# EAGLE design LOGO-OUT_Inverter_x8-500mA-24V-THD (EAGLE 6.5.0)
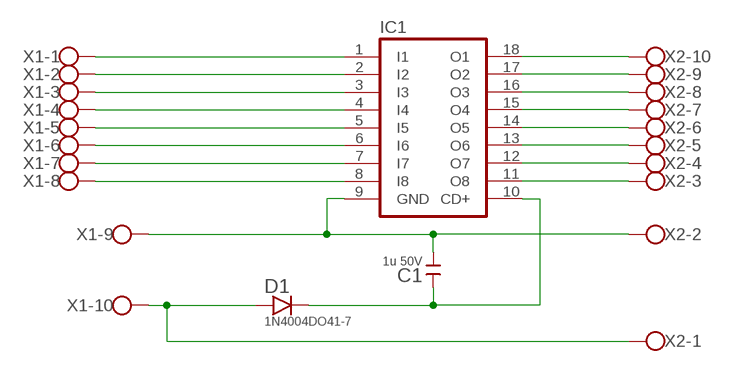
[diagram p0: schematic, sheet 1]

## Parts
C1  1u 50V  C-EU025-024X044  [C025-024X044]
D1  1N4004DO41-7  [DO41-7]
IC1  ULN2803A  [DIL18]
X1  AK500/10  [AK500/10]
X2  AK500/10  [AK500/10]

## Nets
N$1: IC1.1(I1) X1.1
N$2: IC1.2(I2) X1.2
N$3: IC1.3(I3) X1.3
N$4: IC1.4(I4) X1.4
N$5: IC1.5(I5) X1.5
N$6: IC1.6(I6) X1.6
N$7: IC1.7(I7) X1.7
N$8: IC1.8(I8) X1.8
N$9: D1.A X1.10 X2.1
N$10: C1.2 IC1.9(GND) X1.9 X2.2
N$11: IC1.18(O1) X2.10
N$12: IC1.17(O2) X2.9
N$13: IC1.16(O3) X2.8
N$14: IC1.15(O4) X2.7
N$15: IC1.14(O5) X2.6
N$16: IC1.13(O6) X2.5
N$17: IC1.12(O7) X2.4
N$18: IC1.11(O8) X2.3
N$19: C1.1 D1.C IC1.10(CD+)

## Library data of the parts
C1 = rcl:C-EU: CAPACITOR, European symbol
D1 = diode:1N4004: DIODE
IC1 = uln-udn:ULN2803A: DRIVER ARRAY
X1 X2 = con-ptr500:AK500/10: CONNECTOR

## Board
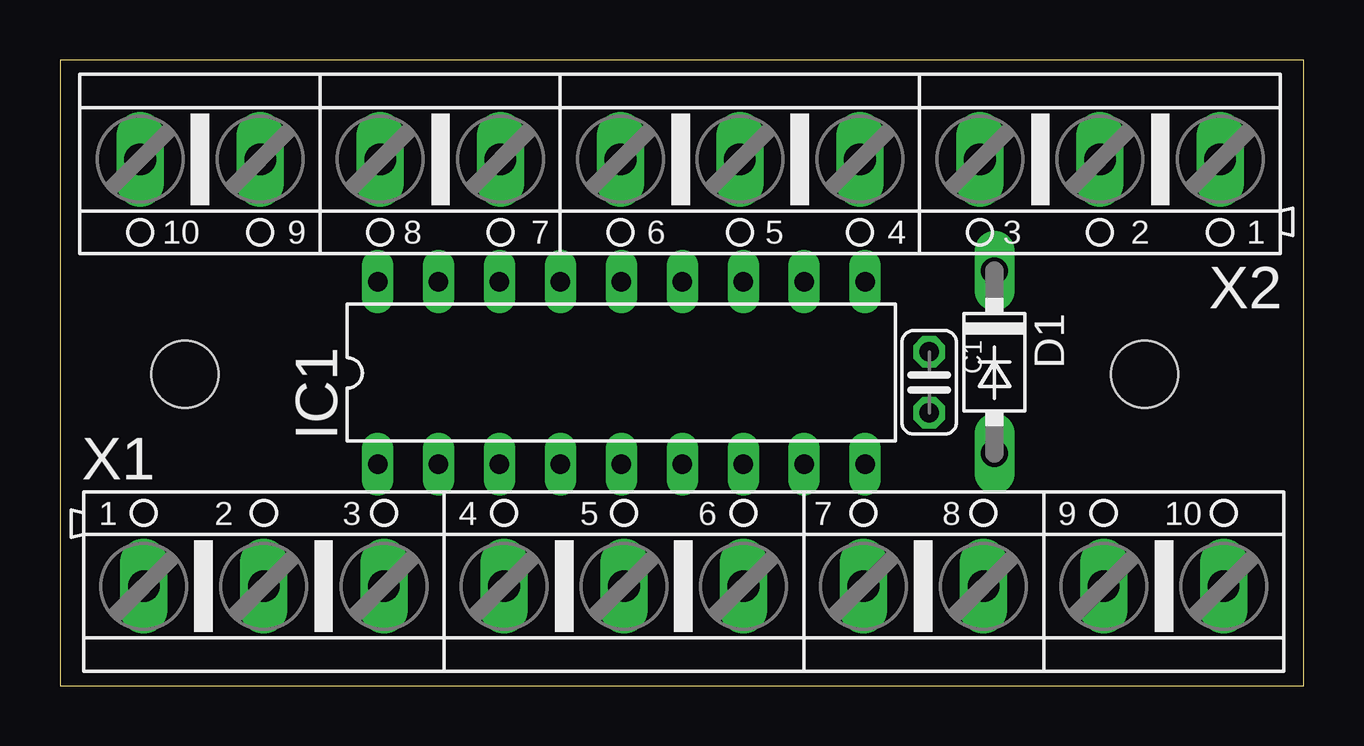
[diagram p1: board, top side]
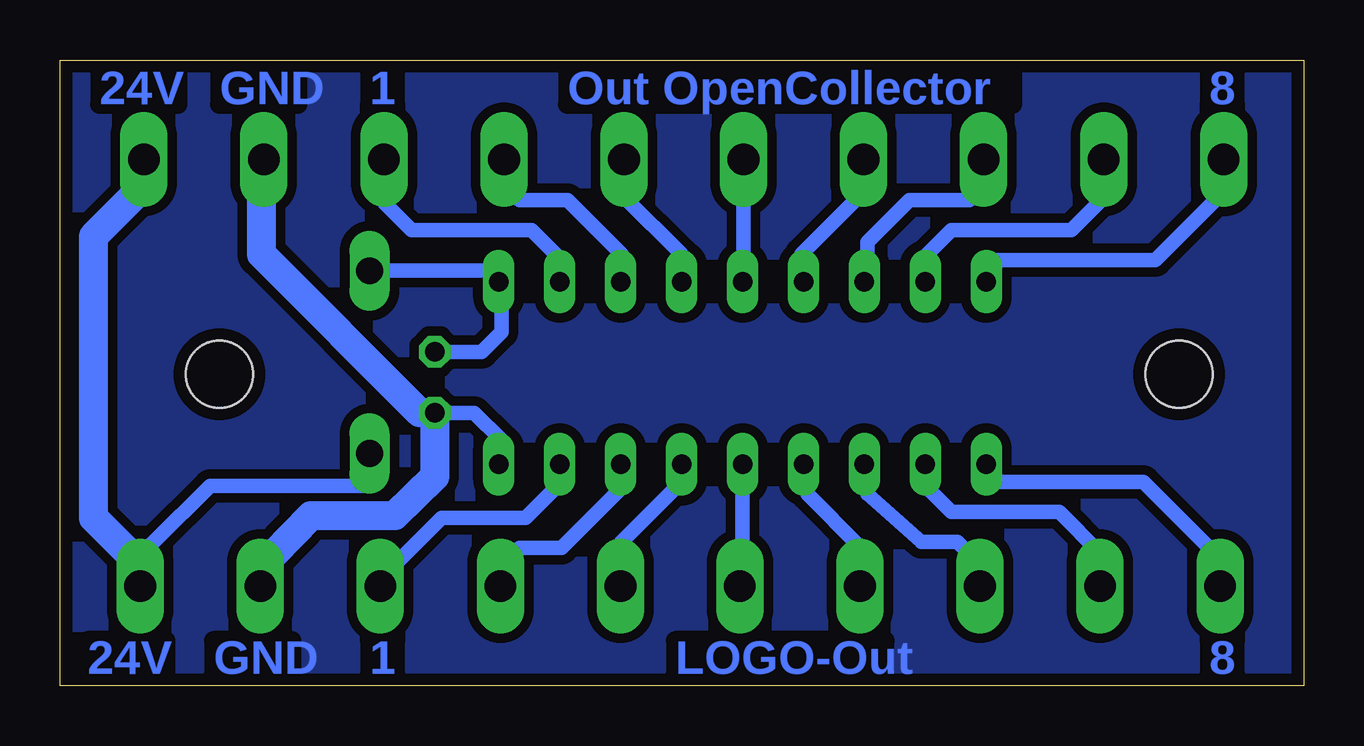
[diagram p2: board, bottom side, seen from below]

Size 51.85 x 26.1 mm. Coordinates in mm from the lower left corner, seen from the top.
Outline: 51.85,0 51.85,26.1 0,26.1 0,0 51.85,0
Copper layers ((1*2)+(15*16)): Top 0.035mm / dielectric 0.7mm / Route2 0.035mm / dielectric 0.15mm / Route15 0.035mm / dielectric 0.7mm / Bottom 0.035mm
Design rules "default *": minimum track width 0.6mm, minimum drill 0.3mm, track to track 0.15mm, track to pad 0.15mm, pad to pad 0.15mm, via to via 0.15mm, smd to smd 2mil, copper to edge 20mil, drill to drill 7mil, minimum pad ring 10mil, minimum via ring 8mil, stop-mask expansion 0.05mm, vias tented up to drill 0.6mm, thermal gap 10mil
Holes 2.8 mm at 5.2,13 45.2,13

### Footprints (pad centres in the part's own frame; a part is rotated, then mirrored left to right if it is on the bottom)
C025-024X044 = drill 0.813 octagon: 1 -1.27,0; 2 1.27,0
DO41-7 = drill 1.118 long: A 3.81,0; C -3.81,0
DIL18 = drill 0.813 long: 1 -10.16,-3.81; 2 -7.62,-3.81; 3 -5.08,-3.81; 4 -2.54,-3.81; 5 0,-3.81; 6 2.54,-3.81; 7 5.08,-3.81; 8 7.62,-3.81; 9 10.16,-3.81; 10 10.16,3.81; 11 7.62,3.81; 12 5.08,3.81; 13 2.54,3.81; 14 0,3.81; 15 -2.54,3.81; 16 -5.08,3.81; 17 -7.62,3.81; 18 -10.16,3.81
AK500/10 = drill 1.321 long: 1 -22.504,0; 2 -17.501,0; 3 -12.497,0; 4 -7.493,0; 5 -2.489,0; 6 2.489,0; 7 7.493,0; 8 12.497,0; 9 17.501,0; 10 22.504,0

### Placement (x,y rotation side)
C1  36.23,12.66 270 top
D1  38.95,13.5 270 top
IC1  23.4,13.05 0 top
X1  26,4.16 0 top
X2  25.85,21.96 180 top

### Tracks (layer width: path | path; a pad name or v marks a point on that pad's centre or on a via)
N$1
  Bottom 0.6: X1.1 3.5,5.3 6.7,8.5 13.25,8.5 IC1.1
N$2
  Bottom 0.6: X1.2 8.5,5.55 10.2,7.25 14.7,7.25 15.7,8.25 15.7,9.16 IC1.2
N$3
  Bottom 0.6: X1.3 13.5,5.05 14.45,6 15.95,6 18.2,8 18.2,9.12 IC1.3
N$4
  Bottom 0.6: X1.4 18.51,5.81 20.7,8 20.7,9.08 IC1.4
N$5
  Bottom 0.6: IC1.5 23.4,4.27 X1.5
N$6
  Bottom 0.6: X1.6 28.49,5.96 25.95,8.5 IC1.6
N$7
  Bottom 0.6: X1.7 33.49,4.96 32.7,5.75 30.95,5.75 28.45,8.25 28.45,9.21 IC1.7
N$8
  Bottom 0.6: IC1.8 31.02,8.43 32.45,7 35.95,7 38.45,4.5 38.45,4.21 X1.8
N$9
  Bottom 0.6: 50.37,18.33 50.45,18.25 | D1.A 38.95,8.5 39.1,8.35 45.6,8.35 47.95,6 48.7,5.25
  Bottom 1.2: X1.10 48.5,5.05 48.7,5.25 50.45,7 50.45,18.25 50.45,18.75 48.45,20.75 48.45,21.86 X2.1
N$10
  Bottom 0.6: C1.2 34.59,11.39 33.45,10.25 33.45,9.35 IC1.9
  Bottom 1.2: X2.2 43.45,21.86 43.45,18 36.84,11.39 C1.2 36.23,8.72 37.9,7.1 41.4,7.1 42.95,5.5 43.45,5 43.45,4.21 X1.9
N$11
  Bottom 0.6: X2.10 3.35,20.6 6.2,17.75 13.2,17.75 13.2,17.15 IC1.18
N$12
  Bottom 0.6: X2.9 8.35,20.35 9.7,19 14.7,19 15.7,18 15.7,16.94 IC1.17
N$13
  Bottom 0.6: X2.8 13.35,20.85 13.95,20.25 16.45,20.25 18.2,18.5 18.2,16.98 IC1.16
N$14
  Bottom 0.6: X2.7 18.36,20.59 20.95,18 20.95,16.95 IC1.15
N$15
  Bottom 0.6: X2.6 23.36,16.9 IC1.14
N$16
  Bottom 0.6: X2.5 28.34,20.39 25.95,18 IC1.13
N$17
  Bottom 0.6: X2.4 33.34,20.89 32.7,20.25 30.7,20.25 28.45,18 28.45,16.89 IC1.12
N$18
  Bottom 0.6: X2.3 38.35,20.15 37.2,19 32.2,19 31.2,18 31.2,17.04 IC1.11
N$19
  Bottom 0.6: C1.1 34.27,13.93 33.45,14.75 33.45,16.75 IC1.10 34.01,17.31 D1.C
N$20
  pour Bottom (isolate 0.4): 0.45,25.5 51.2,25.5 51.2,0.5 0.45,0.5

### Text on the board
Bottom: 8 | Out OpenCollector | 1 | GND | 24V | 8 | LOGO-Out | 1 | GND | 24V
